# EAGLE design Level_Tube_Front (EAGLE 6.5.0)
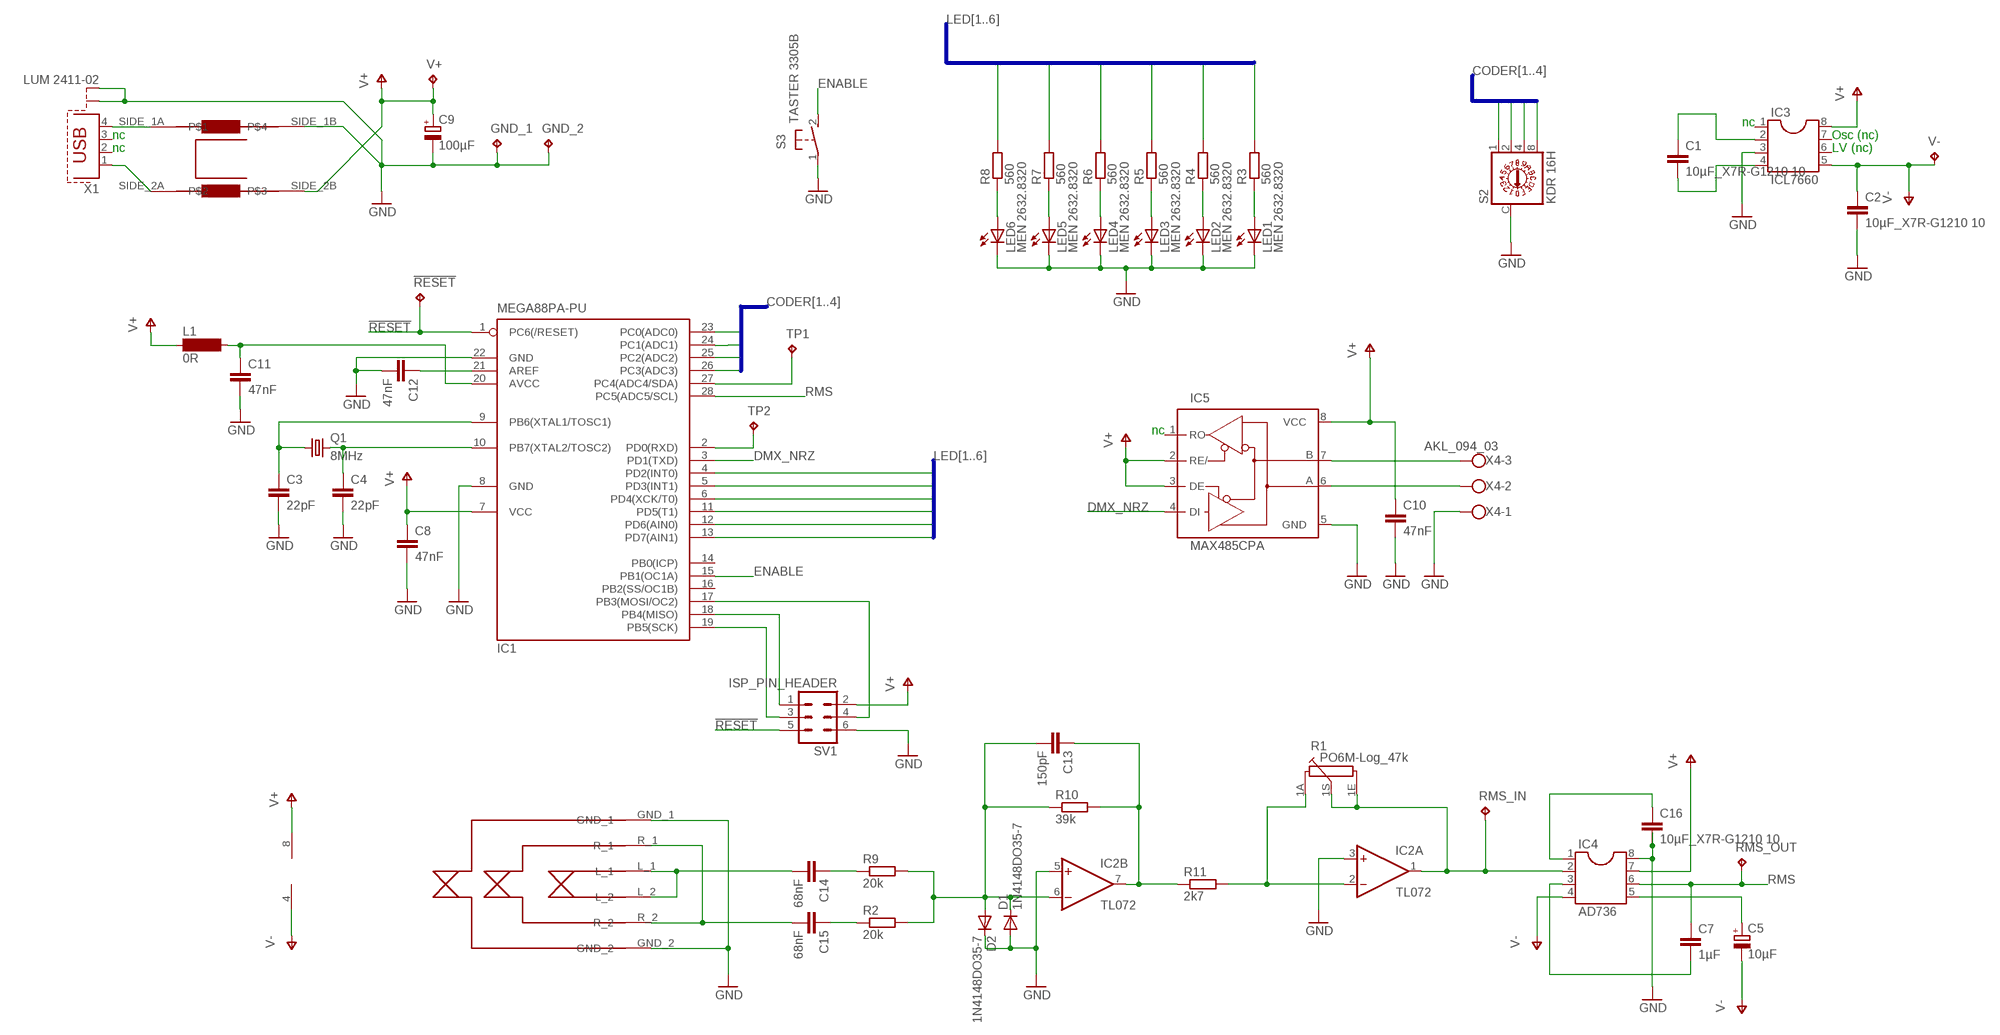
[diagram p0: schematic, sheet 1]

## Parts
!RESET  RTM 1,3-100  TPPAD1-13  [P1-13]
C1  10µF_X7R-G1210 10  C-EUC1206K  [C1206K]
C2  10µF_X7R-G1210 10  C-EUC1206K  [C1206K]
C3  22pF  C-EUC0805  [C0805]
C4  22pF  C-EUC0805  [C0805]
C5  10µF  CPOL-EUE2-5  [E2-5]
C7  1µF  C-EUC1206K  [C1206K]
C8  47nF  C-EUC1206  [C1206]
C9  100µF  CPOL-EUE2-5  [E2-5]
C10  47nF  C-EUC1206  [C1206]
C11  47nF  C-EUC1206  [C1206]
C12  47nF  C-EUC1206  [C1206]
C13  150pF  C-EUC0805  [C0805]
C14  68nF  C-EUC1206K  [C1206K]
C15  68nF  C-EUC1206K  [C1206K]
C16  10µF_X7R-G1210 10  C-EUC1206K  [C1206K]
D1  1N4148DO35-7  [DO35-7]
D2  1N4148DO35-7  [DO35-7]
GND_1  None  TPPAD1-13  [P1-13]
GND_2  RTM 1,3-100  TPPAD1-13  [P1-13]
IC1  MEGA88PA-PU  MEGA8-P  [DIL28-3]
IC2  TL072  TL072P  [DIL08]
IC3  ICL7660  DIL8  [DIL08]
IC4  AD736  DIL8  [DIL08]
IC5  MAX485CPA  MAX3468CPA  [DIL08]
L1  0R  SM-1206  [SM-1206]
LED1  MEN 2632.8320  TLLR4400  [LED3MM]
LED2  MEN 2632.8320  TLLR4400  [LED3MM]
LED3  MEN 2632.8320  TLLR4400  [LED3MM]
LED4  MEN 2632.8320  TLLR4400  [LED3MM]
LED5  MEN 2632.8320  TLLR4400  [LED3MM]
LED6  MEN 2632.8320  TLLR4400  [LED3MM]
Q1  8MHz  CRYSTALHC49S  [HC49/S]
R1  PO6M-Log_47k  PC16S  [PC16S]
R2  20k  R-EU_R1206  [R1206]
R3  560  R-EU_M1206  [M1206]
R4  560  R-EU_M1206  [M1206]
R5  560  R-EU_M1206  [M1206]
R6  560  R-EU_M1206  [M1206]
R7  560  R-EU_M1206  [M1206]
R8  560  R-EU_M1206  [M1206]
R9  20k  R-EU_R1206  [R1206]
R10  39k  R-EU_R1206  [R1206]
R11  2k7  R-EU_R1206  [R1206]
RMS_IN  TPPAD1-13  [P1-13]
RMS_OUT  RTM 1,3-100  TPPAD1-13  [P1-13]
S2  KDR 16H  P103L  [P101L]
S3  TASTER 3305B  31-XX  [B3F-31XX]
SV1  ISP_PIN_HEADER  MA03-2  [MA03-2]
TP1  RTM 1,3-100  TPPAD1-13  [P1-13]
TP2  RTM 1,3-100  TPPAD1-13  [P1-13]
U$1  KLINKENBUCHSE_6.35_EBS_63P  KLINKENBUCHSE_6.35  [STANDARD]
U$2  COMMON_MODE_CHOKE_CAF_0,5-47  COMMON_MODE_CHOKE  [COMMON_MODE]
V+  RTM 1,3-100  TPPAD1-13  [P1-13]
V-  TPPAD1-13  [P1-13]
X1  LUM 2411-02  PN61729-S  [PN61729-S]
X4  AKL_094_03  W237-103  [W237-103]

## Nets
!RESET: !RESET.TP IC1.1(PC6(/RESET)) SV1.5
AVCC: C11.1 IC1.20(AVCC) L1.2
CODER1: IC1.23(PC0(ADC0)) S2.1
CODER2: IC1.24(PC1(ADC1)) S2.2
CODER3: IC1.25(PC2(ADC2)) S2.4
CODER4: IC1.26(PC3(ADC3)) S2.8
DMX_NRZ: IC1.3(PD1(TXD)) IC5.4(DI)
ENABLE: IC1.15(PB1(OC1A)) S3.2(S)
GND: C2.2 C3.2 C4.2 C8.2 C9.- C10.2 C11.2 C12.2 C16.2 D1.A D2.C GND_1.TP GND_2.TP IC1.8(GND) IC1.22(GND) IC2.3(A:+IN) IC2.5(B:+IN) IC3.3 IC4.8 IC5.5(GND) LED1.K(C) LED2.K(C) LED3.K(C) LED4.K(C) LED5.K(C) LED6.K(C) S2.C S3.1(P) SV1.6 U$1.GND_1 U$1.GND_2 U$2.SIDE_1B X1.S1 X1.S2 X4.1
LED1: IC1.13(PD7(AIN1)) R3.2
LED2: IC1.12(PD6(AIN0)) R4.2
LED3: IC1.11(PD5(T1)) R5.2
LED4: IC1.6(PD4(XCK/T0)) R6.2
LED5: IC1.5(PD3(INT1)) R7.2
LED6: IC1.4(PD2(INT0)) R8.2
N$1: IC1.17(PB3(MOSI/OC2)) SV1.4
N$2: C14.2 U$1.L_1 U$1.L_2
N$3: C15.2 U$1.R_1 U$1.R_2
N$4: IC1.18(PB4(MISO)) SV1.1
N$5: LED6.A R8.1
N$6: LED5.A R7.1
N$7: LED4.A R6.1
N$8: LED3.A R5.1
N$9: LED2.A R4.1
N$10: LED1.A R3.1
N$11: IC1.19(PB5(SCK)) SV1.3
N$12: U$2.SIDE_1A X1.4
N$13: C1.2 IC3.4
N$14: C1.1 IC3.2
N$15: C3.1 IC1.9(PB6(XTAL1/TOSC1)) Q1.1
N$16: C4.1 IC1.10(PB7(XTAL2/TOSC2)) Q1.2
N$18: C5.+ IC4.5
N$19: IC2.1(A:OUT) IC4.2 R1.1E R1.1S RMS_IN.TP
N$20: C7.2 IC4.3
N$21: C16.1 IC4.1
N$22: IC5.7(B) X4.3
N$23: C13.2 D1.C D2.A IC2.6(B:-IN) R2.2 R9.2 R10.1
N$24: IC5.6(A) X4.2
N$25: C12.1 IC1.21(AREF)
N$26: IC1.27(PC4(ADC4/SDA)) TP1.TP
N$27: U$2.SIDE_2A X1.1
N$28: IC1.2(PD0(RXD)) TP2.TP
N$29: IC2.2(A:-IN) R1.1A R11.2
N$30: C14.1 R9.1
N$31: C15.1 R2.1
N$32: C13.1 IC2.7(B:OUT) R10.2 R11.1
RMS: C7.1 IC1.28(PC5(ADC5/SCL)) IC4.6 RMS_OUT.TP
V+: C8.1 C9.+ C10.1 IC1.7(VCC) IC2.8(P:V+) IC3.8 IC4.7 IC5.2(RE/) IC5.3(DE) IC5.8(VCC) L1.1 SV1.2 U$2.SIDE_2B V+.TP
V-: C2.1 C5.- IC2.4(P:V-) IC3.5 IC4.4 V-.TP
Unconnected: IC1.14(PB0(ICP)) IC1.16(PB2(SS/OC1B)) IC3.1 IC3.6 IC3.7 IC5.1(RO) X1.2 X1.3

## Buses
LED[1..6]
CODER[1..4]

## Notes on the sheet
- nc
- nc | Osc (nc)
- nc | LV (nc)
- nc

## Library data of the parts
!RESET GND_1 GND_2 RMS_IN RMS_OUT TP1 TP2 V+ V- = testpad:TP: Test pad
C1-C4 C7 C8 C10-C16 = rcl:C-EU: CAPACITOR, European symbol
C5 C9 = rcl:CPOL-EU: POLARIZED CAPACITOR, European symbol
D1 D2 = diode:1N4148: DIODE
IC1 = atmel:MEGA8-P: MICROCONTROLLER 8 Kbytes FLASH, 1 kbytes SRAM, 512 bytes EEPROM, USART, 4-channel 10 bit ADC, 2-channel 8 bit ADC Pin compatible with Atmega48, ATMega88, ATMega168 Source: avr.lbr; OC_FARNELL: unknown; OC_NEWARK: unknown
IC2 = linear:TL072: OP AMP
IC3 IC4 = ic-package:DIL8: Dual In Line / Socket
IC5 = maxim:MAX34*: +5V, Fail-Safe, 40Mbps, Profibus RS-485/RS-422 Transceivers Source: MAX3465-MAX3469.pdf; OC_FARNELL: unknown; OC_NEWARK: unknown
L1 = inductor-neosid:SM-1206: INDUCTOR; OC_FARNELL: unknown; OC_NEWARK: unknown
LED1-LED6 = led:TLLR4400: Low Current (2mA) LED 3 mm Tinted Diffused Package color RED; MF: VISHAY SEMICONDUCTOR; OC_FARNELL: 1612437
Q1 = crystal:CRYSTAL: CRYSTAL; OC_FARNELL: 1667008; OC_NEWARK: unknown
R1 = piher:PC16S: POTENTIOMETER single carbon potentiometer, 16 mm, S3ROH; OC_FARNELL: 4452940; OC_NEWARK: unknown
R2-R11 = rcl:R-EU_: RESISTOR, European symbol
S2 = switch-dil:P103L: DIL/CODE SWITCH; OC_FARNELL: unknown; OC_NEWARK: unknown
S3 = switch-omron:31-XX: OMRON SWITCH; MPN: B3F-3100; OC_FARNELL: 959704; OC_NEWARK: 36M3582
SV1 = con-lstb:MA03-2: PIN HEADER; OC_FARNELL: unknown; OC_NEWARK: unknown
U$1 = leveltube:KLINKENBUCHSE_6.35: Klinkenbuchse für 6.35 mm Neutronik NEUTRIK NR-J6HF
U$2 = leveltube:COMMON_MODE_CHOKE
X1 = con-berg:PN61729-S: BERG USB connector; OC_FARNELL: unknown; OC_NEWARK: unknown
X4 = con-wago-500:W237-103: WAGO SCREW CLAMP; MPN: 237-103; OC_FARNELL: unknown; OC_NEWARK: 18M7116

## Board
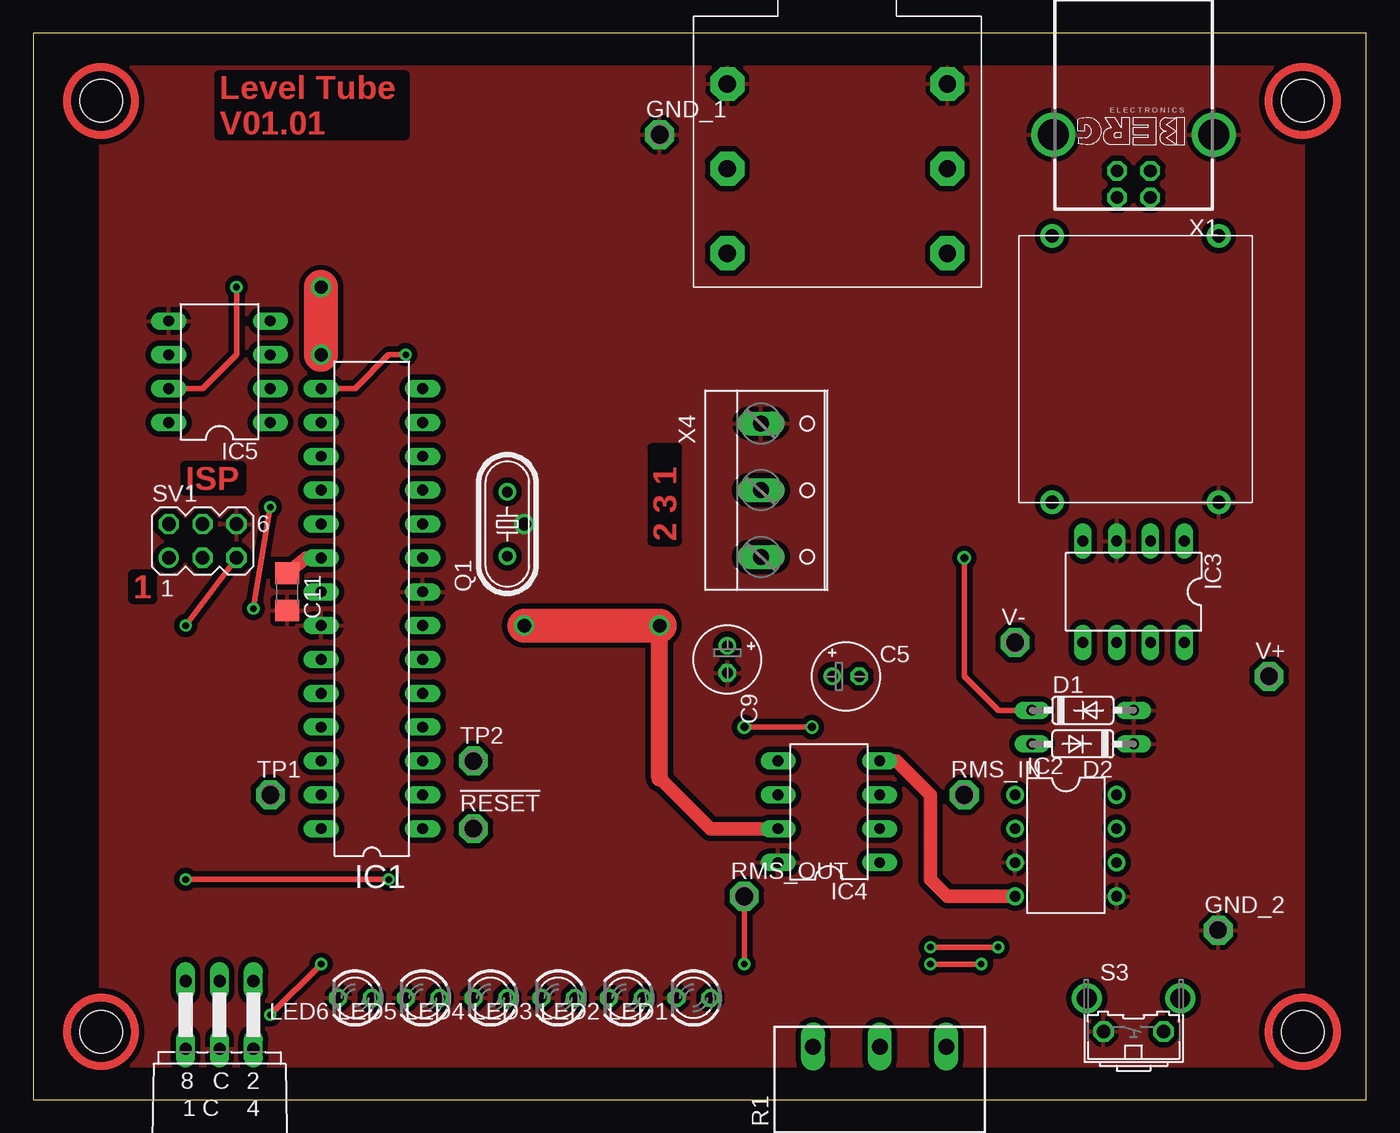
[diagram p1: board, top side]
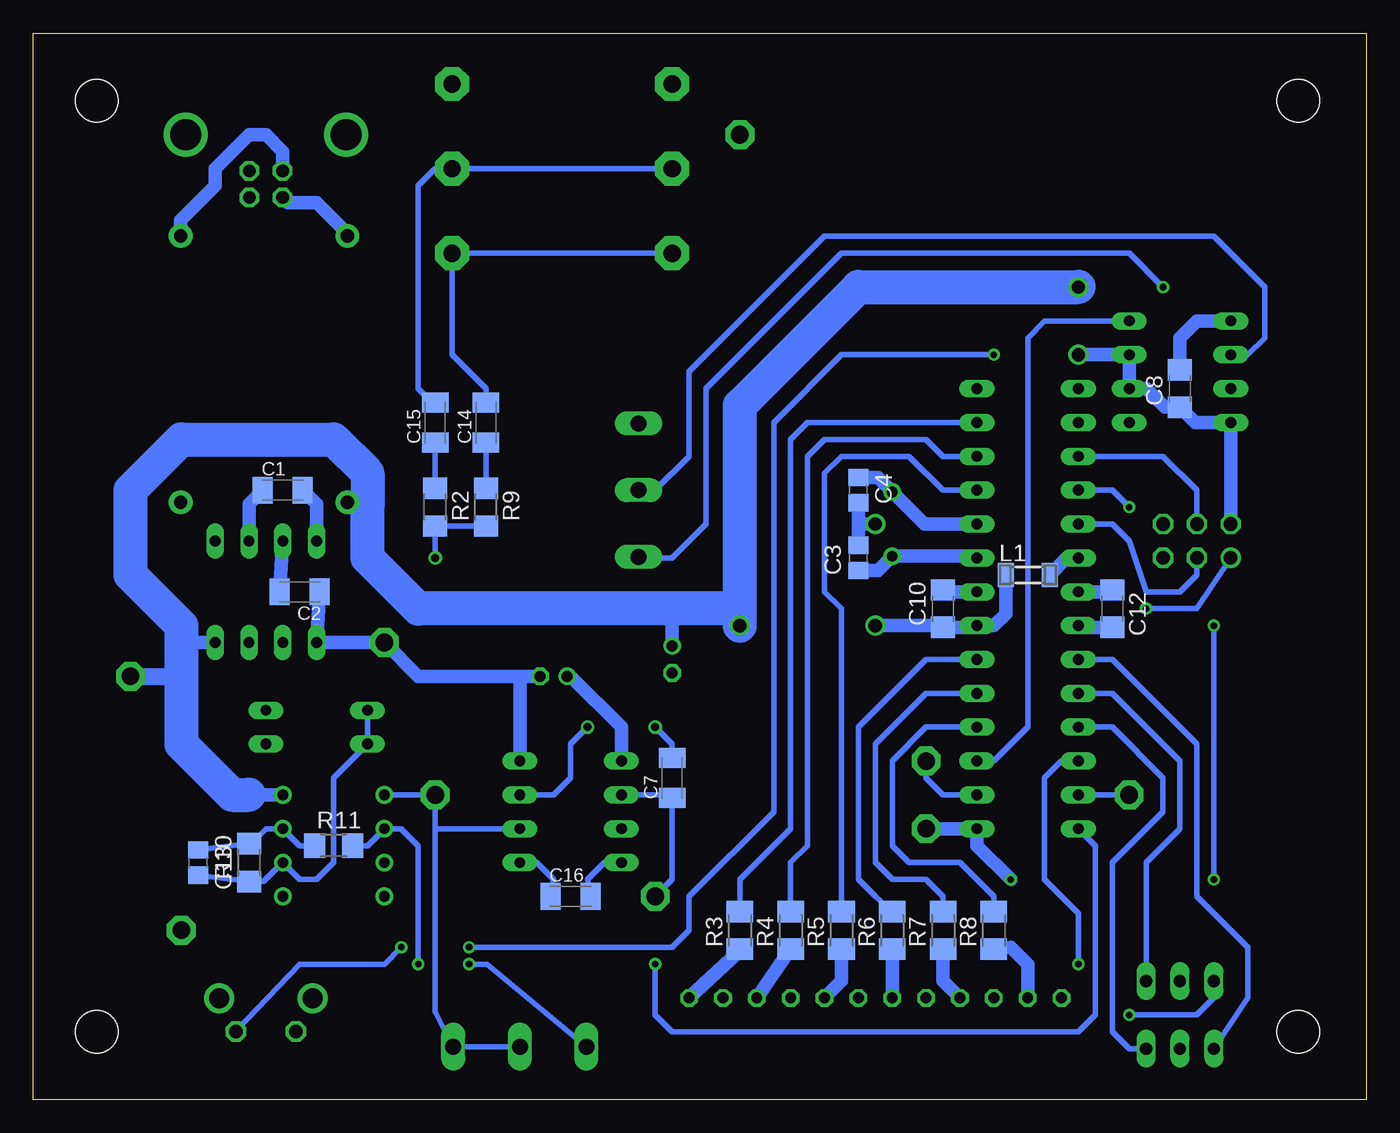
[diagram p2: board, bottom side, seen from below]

Size 100 x 80 mm. Coordinates in mm from the lower left corner, seen from the top.
Outline: 0,0 100,0 100,80 0,80 0,0
Copper layers (1*16): Top 0.035mm / dielectric 1.5mm / Bottom 0.035mm
Design rules "default *": minimum track width 10mil, minimum drill 15mil, track to track 12mil, track to pad 12mil, pad to pad 12mil, via to via 12mil, smd to smd 12mil, copper to edge 1mm, drill to drill 12mil, minimum pad ring 10mil, minimum via ring 8mil, stop-mask expansion 4mil, vias tented up to drill 0mil, thermal gap 15mil
Holes 3.2 mm at 5.08,74.93 5.08,5.08 95.25,5.08 95.25,74.93

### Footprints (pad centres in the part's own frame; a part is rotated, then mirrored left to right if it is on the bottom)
P1-13 = drill 1.321 pad 2.159 octagon: TP 0,0
C1206K = smd 1.5 x 2: 1 -1.5,0; 2 1.5,0
C0805 = smd 1.3 x 1.5: 1 -0.95,0; 2 0.95,0
E2-5 = drill 0.813 pad 1.27: + -1.016,0 | drill 0.813 pad 1.27 octagon: - 1.016,0
C1206 = smd 1.6 x 1.8: 1 -1.4,0; 2 1.4,0
DO35-7 = drill 0.813 long: A 3.81,0; C -3.81,0
DIL28-3 = drill 0.813 long: 1 -16.51,-3.81; 2 -13.97,-3.81; 3 -11.43,-3.81; 4 -8.89,-3.81; 5 -6.35,-3.81; 6 -3.81,-3.81; 7 -1.27,-3.81; 8 1.27,-3.81; 9 3.81,-3.81; 10 6.35,-3.81; 11 8.89,-3.81; 12 11.43,-3.81; 13 13.97,-3.81; 14 16.51,-3.81; 15 16.51,3.81; 16 13.97,3.81; 17 11.43,3.81; 18 8.89,3.81; 19 6.35,3.81; 20 3.81,3.81; 21 1.27,3.81; 22 -1.27,3.81; 23 -3.81,3.81; 24 -6.35,3.81; 25 -8.89,3.81; 26 -11.43,3.81; 27 -13.97,3.81; 28 -16.51,3.81
DIL08 = drill 0.813 pad 1.27: 1 -3.81,-3.81; 2 -1.27,-3.81; 3 1.27,-3.81; 4 3.81,-3.81; 5 3.81,3.81; 6 1.27,3.81; 7 -1.27,3.81; 8 -3.81,3.81
DIL08' = drill 0.813 long: 1 -3.81,-3.81; 2 -1.27,-3.81; 3 1.27,-3.81; 4 3.81,-3.81; 5 3.81,3.81; 6 1.27,3.81; 7 -1.27,3.81; 8 -3.81,3.81
SM-1206 = smd 1.2 x 1.8: 1 -1.65,0; 2 1.65,0
LED3MM = drill 0.813 octagon: A -1.27,0; K 1.27,0
HC49/S = drill 0.813: 1 -2.413,0; 2 2.413,0
PC16S = drill 1.2 long: 1A -5,6.5; 1E 5,6.5; 1S 0,6.5
R1206 = smd 1.6 x 1.803: 1 -1.422,0; 2 1.422,0
M1206 = smd 1.6 x 2: 1 -1.4,0; 2 1.4,0
P101L = drill 0.914 long: 1 -2.54,2.54; 2 2.54,7.62; 4 2.54,2.54; 8 -2.54,7.62; C 0,2.54; C1 0,7.62
B3F-31XX = drill 1.016 octagon: 1 -2.261,-1.245; 2 2.261,-1.245 | drill 1.499 pad 2.159: 3 -3.505,1.245; 4 3.505,1.245
MA03-2 = drill 1.016: 1 -2.54,-1.27 | drill 1.016 octagon: 2 -2.54,1.27; 3 0,-1.27; 4 0,1.27; 5 2.54,-1.27; 6 2.54,1.27
STANDARD = drill 1.3 pad 2.54 octagon: GND_1 2.54,15.24; GND_2 19.05,15.24; L_1 2.54,2.54; L_2 19.05,2.54; R_1 2.54,8.89; R_2 19.05,8.89
COMMON_MODE = drill 1 pad 1.778: SIDE_1A 2.5,2.5; SIDE_1B 2.5,22.5; SIDE_2A 15,2.5; SIDE_2B 15,22.5
PN61729-S = drill 0.95 octagon: 1 1.25,4.71; 2 -1.25,4.71; 3 -1.25,2.71; 4 1.25,2.71 | drill 2.3 pad 2.9: S1 -6.02,0; S2 6.02,0
W237-103 = drill 1.194 long: 1 -5,-1.29; 2 0,-1.29; 3 5,-1.29

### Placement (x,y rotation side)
!RESET  33.02,20.32 0 top
C1  81.28,45.72 0 bottom
C2  80.01,38.1 180 bottom
C3  38.1,40.64 90 bottom
C4  38.1,45.72 270 bottom
C5  60.96,31.75 0 top
C7  52.07,24.13 90 bottom
C8  13.97,53.34 90 bottom
C9  52.07,33.02 270 top
C10  31.75,36.83 90 bottom
C11  19.05,38.1 270 top
C12  19.05,36.83 270 bottom
C13  87.63,17.78 270 bottom
C14  66.04,50.8 90 bottom
C15  69.85,50.8 90 bottom
C16  59.69,15.24 0 bottom
D1  78.74,29.21 0 top
D2  78.74,26.67 180 top
GND_1  46.99,72.39 0 top
GND_2  88.9,12.7 0 top
IC1  25.4,36.83 90 top
IC2  77.47,19.05 270 top
IC3  ICL7660  [DIL08']  82.55,38.1 180 top
IC4  AD736  [DIL08']  59.69,21.59 90 top
IC5  MAX485CPA  [DIL08']  13.97,54.61 90 top
L1  25.4,39.37 0 bottom
LED1  49.53,7.62 180 top
LED2  44.45,7.62 180 top
LED3  39.37,7.62 180 top
LED4  34.29,7.62 180 top
LED5  29.21,7.62 180 top
LED6  24.13,7.62 180 top
Q1  35.56,43.18 90 top
R1  63.5,-2.54 0 top
R2  69.85,44.45 270 bottom
R3  46.99,12.7 90 bottom
R4  43.18,12.7 90 bottom
R5  39.37,12.7 90 bottom
R6  35.56,12.7 90 bottom
R7  31.75,12.7 90 bottom
R8  27.94,12.7 90 bottom
R9  66.04,44.45 270 bottom
R10  83.82,17.78 90 bottom
R11  77.47,19.05 0 bottom
RMS_IN  69.85,22.86 0 top
RMS_OUT  53.34,15.24 0 top
S2  13.97,1.27 0 top
S3  82.55,6.35 0 top
SV1  12.7,41.91 0 top
TP1  17.78,22.86 0 top
TP2  33.02,25.4 0 top
U$1  49.53,60.96 0 top
U$2  91.44,67.31 180 top
V+  92.71,31.75 0 top
V-  73.66,34.29 0 top
X1  82.55,72.39 180 top
X4  55.88,45.72 270 top

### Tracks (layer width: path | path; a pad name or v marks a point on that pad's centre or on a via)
!RESET  (via drill 0.5)
  Top 0.406: v11.43,16.51 v26.67,16.51 | v11.43,35.56 SV1.5
  Bottom 0.406: v11.43,35.56 v11.43,16.51
  Bottom 1.016: !RESET.TP IC1.1 29.21,19.05 v26.67,16.51
AVCC
  Top 1.016: C11.1 20.45,40.64 IC1.20
  Bottom 1.016: 21.46,40.77 IC1.20 22.48,40.64 L1.2
CODER1
  Bottom 0.406: IC1.23 19.05,33.02 12.7,26.67 12.7,15.24 8.89,11.43 8.89,7.62 S2.1
CODER2
  Bottom 0.406: S2.2 16.51,17.78 13.97,20.32 13.97,25.4 19.05,30.48 IC1.24
CODER3
  Bottom 0.406: S2.4 17.78,3.81 19.05,5.08 19.05,17.78 15.24,21.59 15.24,24.13 19.05,27.94 IC1.25
CODER4  (via drill 0.5)
  Top 0.406: v17.78,6.35 v21.59,10.16
  Bottom 0.406: S2.8 11.43,7.62 12.7,6.35 v17.78,6.35 | IC1.26 22.86,25.4 24.13,24.13 24.13,16.51 21.59,13.97 v21.59,10.16
DMX_NRZ
  Bottom 0.406: IC1.3 27.94,25.4 25.4,27.94 25.4,57.15 24.13,58.42 IC5.4
ENABLE  (via drill 0.5)
  Top 0.406: IC1.15 24.13,53.34 26.67,55.88 v27.94,55.88 | v72.39,11.43 v67.31,11.43
  Bottom 0.406: v27.94,55.88 39.37,55.88 44.45,50.8 44.45,21.59 50.8,15.24 50.8,12.7 52.07,11.43 v67.31,11.43 | S3.2 80.01,10.16 73.66,10.16 v72.39,11.43
GND  (via drill 1)
  Bottom 0.406: IC4.8 57.15,17.78 58.42,16.51 C16.2
  Bottom 1.016: IC1.22 21.46,35.43 C12.2 | C8.2 13.97,57.15 12.7,58.42 IC5.5 | IC1.8 31.62,38.1 C10.2 | 38.1,43.18 C4.2 | C3.2 38.1,43.18 | 38.1,43.18 v36.83,43.18 | C2.2 IC3.3
  pour Top (isolate 0.406): 5.08,77.47 95.25,77.47 95.25,2.54 5.08,2.54
LED1
  Bottom 0.406: R3.2 46.99,16.51 43.18,20.32 43.18,49.53 41.91,50.8 IC1.13
LED2
  Bottom 0.406: R4.2 43.18,17.78 41.91,19.05 41.91,48.26 40.64,49.53 33.02,49.53 31.75,48.26 IC1.12
LED3
  Bottom 0.406: R5.2 39.37,36.83 40.64,38.1 40.64,46.99 39.37,48.26 34.29,48.26 31.75,45.72 IC1.11
LED4
  Bottom 0.406: R6.2 36.83,15.24 38.1,16.51 38.1,27.94 33.02,33.02 IC1.6
LED5
  Bottom 0.406: R7.2 31.75,15.24 33.02,16.51 35.56,16.51 36.83,17.78 36.83,26.67 33.02,30.48 IC1.5
LED6
  Bottom 0.406: R8.2 27.94,15.24 30.48,17.78 34.29,17.78 35.56,19.05 35.56,25.4 33.02,27.94 IC1.4
N$1
  Bottom 0.406: SV1.4 12.7,45.72 15.24,48.26 IC1.17
N$2
  Bottom 0.406: U$1.L_1 U$1.L_2 68.58,55.88 66.04,53.34 C14.2
N$3
  Bottom 0.406: U$1.R_1 U$1.R_2 69.85,69.85 71.12,68.58 71.12,53.34 70.08,52.3 C15.2
N$4  (via drill 0.5)
  Top 0.406: v17.78,44.45 v16.51,36.83
  Bottom 0.406: SV1.1 12.7,36.83 v16.51,36.83 | IC1.18 19.05,45.72 v17.78,44.45
N$5
  Bottom 1.016: R8.1 26.67,11.43 25.4,10.16 LED6.A
N$6
  Bottom 1.016: R7.1 31.75,8.89 LED5.A
N$7
  Bottom 1.016: 35.56,11.43 R6.1 LED4.A
N$8
  Bottom 1.016: R5.1 39.37,8.89 LED3.A
N$9
  Bottom 1.016: R4.1 LED2.A
N$10
  Bottom 0.406: R3.1 46.99,11.18 47.12,11.05
  Bottom 1.016: LED1.A 47.12,11.05 46.99,11.43
N$11
  Bottom 0.406: SV1.3 12.7,39.37 13.97,38.1 16.51,38.1 17.78,41.91 19.05,43.18 IC1.19
N$12
  Bottom 1.016: U$2.SIDE_1A 88.94,66 86.36,68.58 86.36,69.85 83.82,72.39 82.55,72.39 81.28,71.12 81.28,69.7 X1.4
N$13
  Bottom 1.016: C1.2 78.74,44.68 IC3.4
N$14
  Bottom 1.016: C1.1 83.82,44.68 IC3.2
N$15
  Bottom 1.016: C3.1 36.64,39.69 Q1.1 29.34,40.77 IC1.9
N$16
  Bottom 1.016: C4.1 36.64,46.67 Q1.2 33.15,43.18 IC1.10
N$18
  Bottom 1.016: IC4.5 55.88,27.94 59.69,31.75 C5.+
N$19
  Bottom 0.406: 69.85,20.32 69.85,6.58 R1.1E R1.1S | 69.85,20.32 RMS_IN.TP IC2.1 | 69.85,20.32 IC4.2
N$20  (via drill 0.6)
  Top 0.406: v53.34,27.94 v58.42,27.94
  Bottom 0.406: v53.34,27.94 52.07,26.67 C7.2 | IC4.3 60.96,22.86 59.69,24.13 59.69,26.67 v58.42,27.94
N$21
  Bottom 0.406: IC4.1 62.23,17.78 60.96,16.51 C16.1
N$22  (via drill 0.5)
  Top 0.406: IC5.7 12.7,53.34 15.24,55.88 v15.24,60.96
  Bottom 0.406: v15.24,60.96 17.78,63.5 39.37,63.5 49.53,53.34 49.53,43.18 52.07,40.64 54.61,40.64 54.61,40.7 X4.3
N$23  (via drill 0.6)
  Top 0.406: v69.85,40.64 69.85,31.75 72.39,29.21 D1.C
  Bottom 0.406: C13.2 R10.1 82.7,16.36 IC2.6 80.01,16.51 78.74,16.51 77.47,17.78 77.47,24.13 D2.A D1.C | R9.2 R2.2 v69.85,40.64
N$24
  Bottom 0.406: IC5.6 8.89,55.88 7.62,57.15 7.62,60.96 11.43,64.77 40.64,64.77 50.8,54.61 50.8,48.26 53.34,45.72 X4.2
N$25
  Bottom 1.016: C12.1 19.18,38.1 IC1.21
N$26
  Bottom 0.406: TP1.TP IC1.27
N$27
  Bottom 1.016: U$2.SIDE_2A 76.44,65.01 78.74,67.31 80.93,67.31 X1.1
N$28
  Bottom 0.406: IC1.2 31.75,22.86 33.02,24.13 TP2.TP
N$29  (via drill 0.5)
  Top 0.406: v67.31,10.16 v71.12,10.16
  Bottom 0.406: R1.1A 65.97,10.16 v67.31,10.16 | v71.12,10.16 71.12,19.05 72.39,20.32 IC2.2 74.93,19.05 R11.2
N$30
  Bottom 0.406: R9.1 C14.1
N$31
  Bottom 0.406: R2.1 C15.1
N$32
  Bottom 0.406: 83.82,19.05 83.67,19.2 | R11.1 80.01,19.05 IC2.7 82.55,20.32 83.67,19.2 | C13.1 R10.2 83.67,19.2
RMS  (via drill 0.5)
  Top 0.406: v53.34,10.16 RMS_OUT.TP
  Bottom 0.406: IC1.28 20.32,19.05 20.32,6.35 21.59,5.08 52.07,5.08 53.34,6.35 v53.34,10.16 | C7.1 52.07,22.86 | IC4.6 52.3,22.86 C7.1 | C7.1 52.07,16.51 RMS_OUT.TP
V+  (via drill 1)
  Top 1.016: IC4.7 50.8,20.32 46.99,24.13
  Top 1.27: 46.99,24.13 v46.99,35.56
  Top 2.54: v36.83,35.56 v46.99,35.56 | v21.59,55.88 v21.59,60.96
  Bottom 1.016: L1.1 27.05,36.45 27.94,35.56 IC1.7 29.34,35.43 C10.1 31.75,35.56 v36.83,35.56 | SV1.2 IC5.8 12.83,50.8 C8.1 15.11,51.94 16.51,53.34 IC5.2 IC5.3 v21.59,55.88 | 83.82,22.86 IC2.8 | IC3.8 88.9,34.29 | C9.+ 52.07,36.83 | 74.93,44.45 U$2.SIDE_2B
  Bottom 1.27: V+.TP 88.9,31.75
  Bottom 2.54: 46.99,36.83 46.99,52.07 38.1,60.96 v21.59,60.96 | 83.82,22.86 85.09,22.86 88.9,26.67 88.9,31.75 88.9,34.29 88.9,35.56 92.71,39.37 92.71,45.72 88.9,49.53 77.47,49.53 74.93,46.99 74.93,44.45 74.93,40.64 71.12,36.83 52.07,36.83 46.99,36.83 | v46.99,35.56 46.99,36.83
V-
  Top 1.016: IC2.4 68.58,15.24 67.31,16.51 67.31,22.86 64.77,25.4 IC4.4
  Bottom 1.016: 63.5,31.75 IC4.4 | 63.5,31.75 C5.- | 63.5,31.75 71.12,31.75 V-.TP IC3.5 C2.1
(copper drawn outside any net)
  shapes: Top circle x4

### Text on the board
Top: Level Tube / V01.01 | ISP | 2 3 1 | 1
